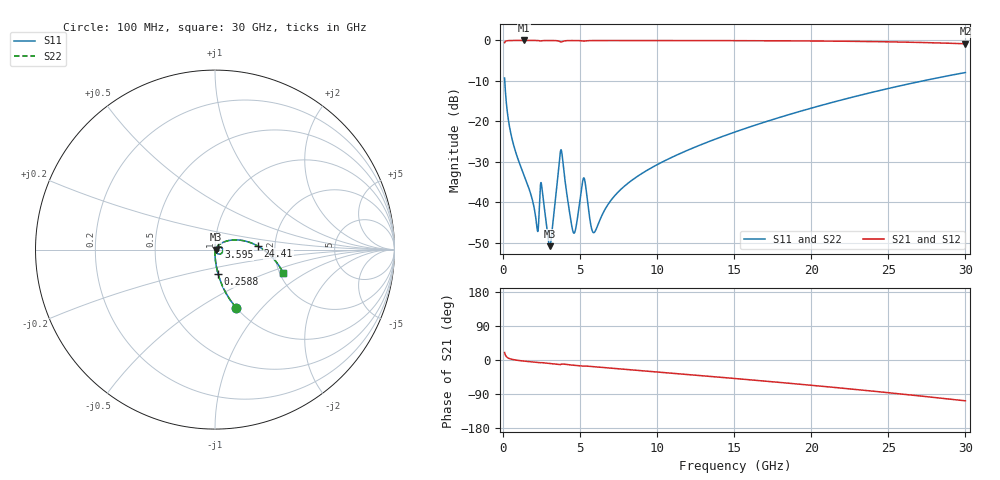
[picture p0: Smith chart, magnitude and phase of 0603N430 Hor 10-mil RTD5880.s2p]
# GHz S MA R 50
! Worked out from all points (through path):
!   3201 points, 100 MHz to 30 GHz, reference 50 ohm
!   highest |S21| = -0.01 dB at 1.38 GHz (marker M1); lowest = -0.8 dB at 30 GHz (marker M2)
!   group delay of S21, straight-line fit = 10 ps
!   lowest |S11| = -50.8 dB at 3.034 GHz (marker M3), VSWR 1.01, Z = 50.3 - j0.059 ohm
!   |S11| at or under -10 dB: 109.6 MHz to 27.24 GHz (27.13 GHz wide, 198 % of centre)
!   |S22| runs from -50.8 to -7.9 dB; largest |S21 - S12| = 0
!   S11 on the Smith chart (normalised r, x): 100 MHz: 1.00, -0.73; 258.8 MHz: 1.00, -0.28; 3.595 GHz: 1.04, +0.03; 24.41 GHz: 1.63, +0.07; 30 GHz: 2.09, -0.64
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0.1  0.3433 -70.2  0.9389 19.8  0.9389 19.8  0.3433 -70.2
0.2588437  0.1391 -82.6  0.9898 7.2  0.9898 7.2  0.1391 -82.6
0.6325937  0.05546 -88.0  0.9977 1.3  0.9977 1.3  0.05546 -88.0
1.380094  0.02113 -90.0  0.9986 -3.0  0.9986 -3.0  0.02113 -90.0
2.183656  0.005165 -66.0  0.9973 -6.4  0.9973 -6.4  0.005165 -66.0
2.538719  0.01416 -61.0  0.9916 -7.1  0.9916 -7.1  0.01416 -61.0
3.033937  0.002868 -11.8  0.9971 -9.2  0.9971 -9.2  0.002868 -11.8
3.594562  0.02488 39.2  0.9842 -12.0  0.9842 -12.0  0.02488 39.2
3.828156  0.03909 -37.0  0.9648 -10.6  0.9648 -10.6  0.03909 -37.0
4.575656  0.004183 -22.2  0.9958 -13.8  0.9958 -13.8  0.004183 -22.2
4.762531  0.005311 17.0  0.9954 -14.6  0.9954 -14.6  0.005311 17.0
5.089563  0.01466 24.2  0.9887 -16.0  0.9887 -16.0  0.01466 24.2
5.304469  0.01859 -23.8  0.9815 -15.9  0.9815 -15.9  0.01859 -23.8
5.696906  0.005202 -30.2  0.9948 -17.2  0.9948 -17.2  0.005202 -30.2
5.921156  0.004243 6.0  0.996 -18.0  0.996 -18.0  0.004243 6.0
7.406813  0.01302 53.9  0.9969 -23.1  0.9969 -23.1  0.01302 53.9
10.06978  0.02964 51.9  0.9962 -31.9  0.9962 -31.9  0.02964 51.9
15.05  0.07387 38.1  0.9931 -48.8  0.9931 -48.8  0.07387 38.1
20.03956  0.1463 21.2  0.984 -66.8  0.984 -66.8  0.1463 21.2
24.41244  0.2399 4.7  0.9646 -83.9  0.9646 -83.9  0.2399 4.7
25.01978  0.2552 2.3  0.9605 -86.4  0.9605 -86.4  0.2552 2.3
30  0.4011 -18.8  0.9084 -107.7  0.9084 -107.7  0.4011 -18.8
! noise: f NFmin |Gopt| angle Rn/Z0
0.1  0.0002923  0.9185  0.3799  0.0007922
3.417  0.006592  0.8793  10.37  0.01172
6.743  0.006642  0.7778  20.37  0.005931
10.06  0.008335  0.7437  30.14  0.006097
13.39  0.01032  0.7304  39.71  0.006766
16.7  0.01234  0.7243  48.97  0.007396
20.03  0.01444  0.7228  57.94  0.00797
23.35  0.01665  0.7249  66.56  0.008492
26.67  0.01903  0.7298  74.88  0.00897
30  0.02164  0.737  82.88  0.009412
